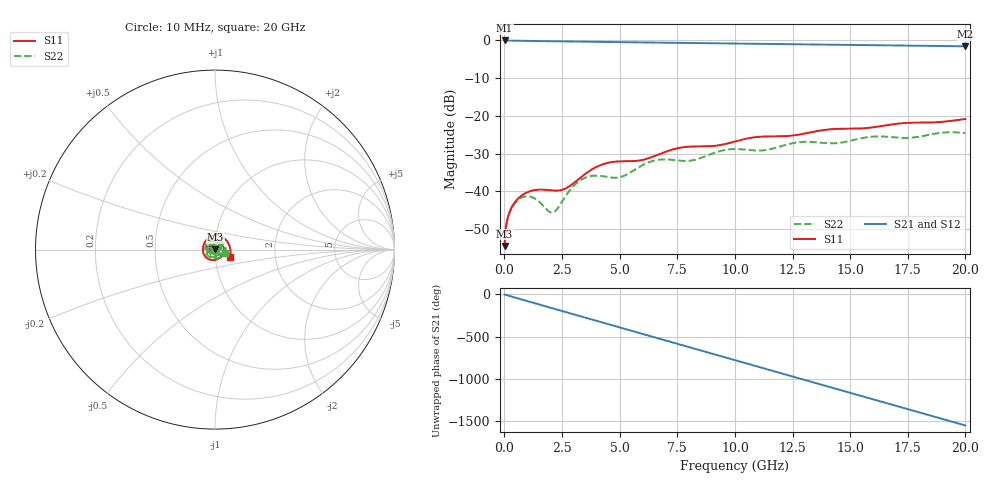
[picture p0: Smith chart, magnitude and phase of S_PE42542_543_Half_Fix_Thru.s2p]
! Peregrine Semiconductor
! File: S_PE42542_543_Half_Fix_Thru.s2p
! For use in vector de-embedding Evaluation Sample Kit s-parameter measurements
! Please refer to Application Note AN39 for further information regarding de-embedding
! Port Definition
!	Port 1 = SMA connectorized port
!	Port 2 = end of PCB transmission line at DUT interface (the exact center of PCB Thru Line)
! Frequency start,  stop,  step,  npts
!  10MHz, 20.0GHz, 24.9875MHz, 801
! freq dB(S11) phase(S11) dB(S12) phase(S12) dB(S21) phase(S21) dB(S22) phase(S22)
#  Hz  S  DB  R 50
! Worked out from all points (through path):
!   801 points, 10 MHz to 20 GHz, reference 50 ohm
!   highest |S21| = -0.02 dB at 10 MHz (marker M1); lowest = -1.6 dB at 20 GHz (marker M2)
!   group delay of S21, straight-line fit = 215 ps
!   lowest |S11| = -54.5 dB at 10 MHz (marker M3), VSWR 1.00, Z = 50.2 + j0.0756 ohm
!   |S11| at or under -10 dB: start of sweep to end of sweep
!   |S22| runs from -54.6 to -24.3 dB; largest |S21 - S12| = 0
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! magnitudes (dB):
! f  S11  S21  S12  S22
! 10 MHz  -54.5  0.0  0.0  -54.6
! 134.9 MHz  -47.3  0.0  0.0  -47.5
! 234.9 MHz  -45.3  -0.1  -0.1  -45.6
! 434.8 MHz  -43.1  -0.1  -0.1  -43.4
! 709.6 MHz  -41.3  -0.1  -0.1  -41.8
! 1.234 GHz  -39.8  -0.2  -0.2  -41.6
! 2.109 GHz  -39.8  -0.2  -0.2  -45.6
! 2.659 GHz  -39.2  -0.3  -0.3  -41.2
! 3.358 GHz  -36.1  -0.3  -0.3  -36.9
! 4.183 GHz  -33.0  -0.4  -0.4  -35.9
! 5.032 GHz  -32.1  -0.5  -0.5  -36.2
! 5.907 GHz  -31.8  -0.5  -0.5  -33.4
! 6.682 GHz  -30.3  -0.6  -0.6  -31.7
! 8.106 GHz  -28.1  -0.7  -0.7  -31.9
! 10.01 GHz  -26.8  -0.8  -0.8  -28.8
! 11.23 GHz  -25.5  -0.9  -0.9  -29.1
! 12.6 GHz  -25.1  -1.0  -1.0  -27.1
! 13.35 GHz  -24.3  -1.1  -1.1  -26.9
! 14.38 GHz  -23.5  -1.2  -1.2  -27.3
! 15.83 GHz  -23.2  -1.3  -1.3  -25.6
! 16.68 GHz  -22.4  -1.3  -1.3  -25.6
! 20 GHz  -20.8  -1.6  -1.6  -24.6
